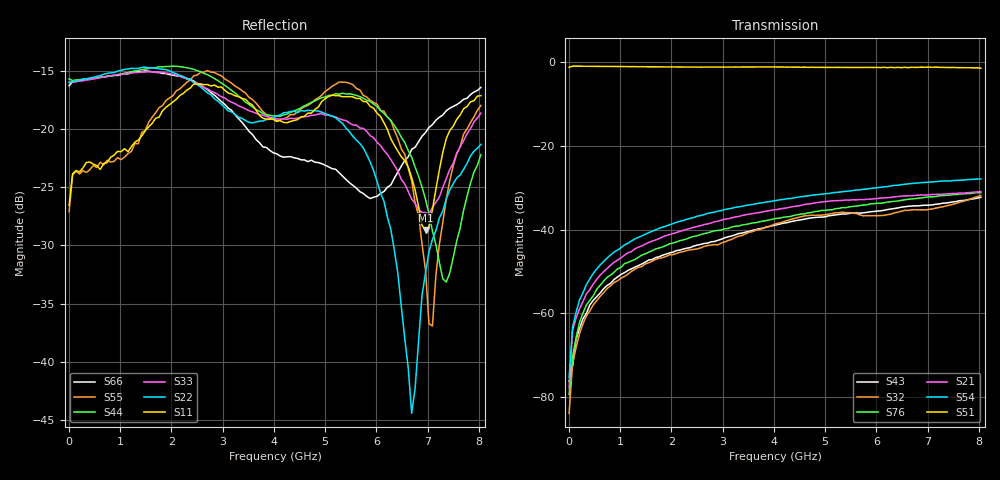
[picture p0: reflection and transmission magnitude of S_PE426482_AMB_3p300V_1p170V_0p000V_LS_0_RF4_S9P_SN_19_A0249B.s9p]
! Device ID: PE426482
! File Path: z:\PE426482\Final Char Data\room\AMB\3p300\LS_0_RF4\PE426482_AMB_3p300V_1p170V_0p000V_LS_0_RF4_S9P_SN_19_A0249B.s9p
! Serial: 19
! Lot: A0249B
! Temp: AMB
! VDD: 3.300
! VSS: 0.000
! Control_Hi: 1.170
! Control_Lo: 0.000
! Logic State: LS_0_RF4
! Port 1:
! Port 2:
! Port 3:
! Port 4:
! Port 5:
! Port 6:
! Port 7:
! Port 8:
! Port 9:
! ThroughPath:1-5
! IDD: 0.0001086967
! ISS/IDD2: -1.43e-008
! IDMM3/IDD3: -2.002e-007
! Comment:
#  Hz  S  RI  R  50
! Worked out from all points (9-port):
!   120 points, 10 MHz to 8.037 GHz, reference 50 ohm
!   strongest paths, dB at 10 MHz, 2.034 GHz, 4.057 GHz, 6.08 GHz, 8.037 GHz:
!     S51: -1.2, -1.1, -1.1, -1.3, -1.4
!     S54: -75.3, -38.6, -33.0, -29.9, -27.9
!     S21: -77.8, -40.9, -35.2, -32.5, -30.9
!     S76: -79.4, -43.2, -37.3, -33.7, -31.2
!     S32: -83.9, -46.0, -38.5, -36.6, -31.8
!     S43: -76.2, -45.4, -38.9, -35.5, -32.3
!   lowest |S11| = -28.7 dB at 6.957 GHz (marker M1), VSWR 1.08, Z = 53.6 + j1.2 ohm
!   |S11| at or under -10 dB: start of sweep to end of sweep
